|   Microchip Technology Inc.
|   PolarFire IBIS Model
[IBIS ver]   5.0
[File name]   polarfire_gpio_se.ibs
[File Rev]   2.3
[Date]   Wed Nov 22 2023
[Source] Simulated Models ONLY.
   All data is based on Spice simulation. All performed at Microchip Technology Inc.
[Notes]   This IBIS file is for GPIO single ended standards.
   Please refer to polarfire_gpio_diff.ibs for GPIO differential Standards Configurations,
   and refer to polarfire_hsio_se.ibs and polarfire_hsio_diff.ibs for HSIO Configurations.
   The package parasitics of various package types are given.
   Uncomment the appropriate package before simulations
   Revision History
   Rev 2.3: 22-Nov-2023
   - Added mixed mode receiver support:
   - Input buffers: LVCMOS12_15_CL_ODT-120,LVCMOS12_18_CL_ODT-120,LVCMOS12_25_CL_ODT-120,
   LVCMOS12_15_CL_ODT-240,LVCMOS12_18_CL_ODT-240,LVCMOS12_25_CL_ODT-240,
   LVCMOS18_15_ODT-120,LVCMOS18_25_ODT-120,LVCMOS18_15_ODT-240,LVCMOS18_25_ODT-240,
   HSUL18_33_ODT-OFF,HSUL18_25_ODT-OFF,HSUL18_15_ODT-OFF,HSUL18_12_ODT-OFF,
   HSUL18_ODT-OFF,HSUL18_ODT-50
   Rev 2.2: 26-Jul-2022
   - Vmeas_rising and Vmeas_falling of pci driver updated for more accuracy
   Rev 2.1: 4-May-2022
   - Vref_falling max voltage updated for pci driver
   - Added MPF050 device with RLC package data in [Package] section
   - Added RLC package type of FCG784N for MPF300T/TS device
   - Update RLC values of 200T-FCVG484 device package data
[Disclaimer] This information is for board design considerations.
   Simulation based V/I curves contained in this model file are
   considered preliminary until verified against bench
   measurements. Maximum currents may vary from part to part but
   should not exceed maximum I/V curves provided in this model file.
[Copyright]  (c) 2023, Microchip Technology Inc., All Rights Reserved.
| ADDITIONAL NOTES
|For Low Power Mobile Industry Processor Interface (MIPI) configuration,please use LVCMOS12 receiver IBIS models.
|Warnings for ISSO Pullup, Pulldown currents being non-zero maybe ignored.
|The naming conventions used in the signal_name/model_name are as follows:
| SLEW-#  - Slew setting,OFF or ON represented by #
| HYST-#  - Hysteresis setting,OFF or ON represented by #
| #mA   - Driver current strength, value represented by #
| #ohm   - Driver impedance mode, value represented by #
| ODT-#   - Series on-die termination, impedance value represented by #
| CL   - Receiver standards with clamp ON
| C1   - Refers to Class-I driver models
| C2   - Refers to Class-II driver models
| #_I   - Refers to input models ,  model name represented by #
| #_O   - Refers to output models , model name represented by #
| IBIS MODEL CHECKLIST
| Microchip Technology Inc. is dedicated to releasing quality IBIS models to customers.
| The following items have been
| verified for this IBIS model before release:
| 1)  Checked IBIS model by the golden parser ibischk5 [Complete]
| 2)  Ensured no errors reported by golden parser
|   for the IBIS model [Complete]
| 3)  Defined Vinl and Vinh for receivers [Complete]
| 4)  Defined Standard Load and Vmeas values for drivers [Complete]
| 5)  Defined overshoots for drivers and receivers [NA]
| 6)  Validated Ramp Values[]
| 7)  Defined V-T Tables for all output drivers [Complete]
| 8)  Validated [Diff Pins] [NA]
| 9)  Verified Package Parasitics [Complete]
| 10) Defined Standard Load Parameters and Specifications
|   for waveforms [Complete]
| 11) Defined and Validate Pin mappings [Complete]
| 12) Verified C_comp_pullup and C_comp_pulldown Values []
| 13) Visually Inspected I-V Curves and V-T Tables  [Complete]
| 14) Presented Typ/Min/Max Values in the correct order for
|   all tables and parameters [Complete]
| 15) Simulated all output models with standard load and
|   switching through Vmeas [Complete]
| 16) Simulated all receiver models  [Complete]
| 17) Validated Models selectors. [NA]
| 18) Visually inspected Spice and IBIS correlation for
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[Component]   PolarFire
[Manufacturer]   Microchip Technology Inc.
[Package]
|   typ   min   max
|MPF050T/TL/TLS/TS
|R_pkg   0.342   NA   NA   | MPF050T/TL/TLS/TS-FCSG325
|L_pkg   2.917nH   NA   NA   | MPF050T/TL/TLS/TS-FCSG325
|C_pkg   1.401pF   NA   NA   | MPF050T/TL/TLS/TS-FCSG325
|R_pkg   0.668   NA   NA   | MPF050T/TL/TLS/TS-FCVG484
|L_pkg   4.858nH   NA   NA   | MPF050T/TL/TLS/TS-FCVG484
|C_pkg   1.717pF   NA   NA   | MPF050T/TL/TLS/TS-FCVG484
|MPF100T/TL/TLS/TS
|R_pkg   0.277   NA   NA   | MPF100T/TL/TLS/TS-FCSG325
|L_pkg   2.866nH   NA   NA   | MPF100T/TL/TLS/TS-FCSG325
|C_pkg   0.601pF   NA   NA   | MPF100T/TL/TLS/TS-FCSG325
|R_pkg   0.960   NA   NA   | MPF100T/TL/TLS/TS-FCG484
|L_pkg   6.090nH   NA   NA   | MPF100T/TL/TLS/TS-FCG484
|C_pkg   2.182pF   NA   NA   | MPF100T/TL/TLS/TS-FCG484
|R_pkg   0.639   NA   NA   | MPF100T/TL/TLS/TS-FCVG484
|L_pkg   4.241nH   NA   NA   | MPF100T/TL/TLS/TS-FCVG484
|C_pkg   1.595pF   NA   NA   | MPF100T/TL/TLS/TS-FCVG484
|MPF200T/TL/TLS/TS
|R_pkg   0.392   NA   NA   | MPF200T/TL/TLS/TS-FCSG325
|L_pkg   3.035nH   NA   NA   | MPF200T/TL/TLS/TS-FCSG325
|C_pkg   0.970pF   NA   NA   | MPF200T/TL/TLS/TS-FCSG325
|R_pkg   0.885   NA   NA   | MPF200T/TL/TLS/TS-FCG484
|L_pkg   5.836nH   NA   NA   | MPF200T/TL/TLS/TS-FCG484
|C_pkg   2.013pF   NA   NA   | MPF200T/TL/TLS/TS-FCG484
|R_pkg   0.634   NA   NA   | MPF200T/TL/TLS/TS-FCVG484
|L_pkg   4.221nH   NA   NA   | MPF200T/TL/TLS/TS-FCVG484
|C_pkg   1.605pF   NA   NA   | MPF200T/TL/TLS/TS-FCVG484
|R_pkg   0.483   NA   NA   | MPF200T/TL/TLS/TS-FCSG536
|L_pkg   4.073nH   NA   NA   | MPF200T/TL/TLS/TS-FCSG536
|C_pkg   1.335pF   NA   NA   | MPF200T/TL/TLS/TS-FCSG536
|R_pkg   1.512   NA   NA   | MPF200T/TL/TLS/TS-FCG784
|L_pkg   9.182nH   NA   NA   | MPF200T/TL/TLS/TS-FCG784
|C_pkg   3.029pF   NA   NA   | MPF200T/TL/TLS/TS-FCG784
|MPF300T/TL/TLS/TS
|R_pkg   0.678   NA   NA   | MPF300T/TL/TLS/TS-FCG484
|L_pkg   5.038nH   NA   NA   | MPF300T/TL/TLS/TS-FCG484
|C_pkg   1.584pF   NA   NA   | MPF300T/TL/TLS/TS-FCG484
|R_pkg   0.702   NA   NA   | MPF300T/TL/TLS/TS-FCVG484
|L_pkg   4.503nH   NA   NA   | MPF300T/TL/TLS/TS-FCVG484
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R_pkg   1.478   NA   NA   | MPF300T/TL/TLS/TS-FCG1152
L_pkg   8.879nH   NA   NA   | MPF300T/TL/TLS/TS-FCG1152
C_pkg   2.839pF   NA   NA   | MPF300T/TL/TLS/TS-FCG1152
|MPF500T/TL/TLS/TS
|R_pkg   1.081   NA   NA   | MPF500T/TL/TLS/TS-FCG784
|L_pkg   6.727nH   NA   NA   | MPF500T/TL/TLS/TS-FCG784
|C_pkg   2.413pF   NA   NA   | MPF500T/TL/TLS/TS-FCG784
|R_pkg   1.419   NA   NA   | MPF500T/TL/TLS/TS-FCG1152
|L_pkg   8.917nH   NA   NA   | MPF500T/TL/TLS/TS-FCG1152
|C_pkg   2.924pF   NA   NA   | MPF500T/TL/TLS/TS-FCG1152
| End Header
| The PIN numbers given below are examples. They do not correspond to
| device pin numbers.
[Pin]   signal_name   model_name   R_pin   L_pin   C_pin
1   PCI_20mA_SLEW-ON_O   PCI_20mA_SLEW-ON_GPIO_O
2   PCI_20mA_SLEW-OFF_O   PCI_20mA_SLEW-OFF_GPIO_O
3   LVTTL_8mA_SLEW-ON_O   LVTTL_8mA_SLEW-ON_GPIO_O
4   LVTTL_8mA_SLEW-OFF_O   LVTTL_8mA_SLEW-OFF_GPIO_O
5   LVTTL_2mA_SLEW-ON_O   LVTTL_2mA_SLEW-ON_GPIO_O
6   LVTTL_2mA_SLEW-OFF_O   LVTTL_2mA_SLEW-OFF_GPIO_O
7   LVTTL_4mA_SLEW-ON_O   LVTTL_4mA_SLEW-ON_GPIO_O
8   LVTTL_4mA_SLEW-OFF_O   LVTTL_4mA_SLEW-OFF_GPIO_O
9   LVTTL_12mA_SLEW-ON_O   LVTTL_12mA_SLEW-ON_GPIO_O
10   LVTTL_12mA_SLEW-OFF_O   LVTTL_12mA_SLEW-OFF_GPIO_O
11   LVTTL_16mA_SLEW-ON_O   LVTTL_16mA_SLEW-ON_GPIO_O
12   LVTTL_16mA_SLEW-OFF_O   LVTTL_16mA_SLEW-OFF_GPIO_O
13   LVTTL_20mA_SLEW-ON_O   LVTTL_20mA_SLEW-ON_GPIO_O
14   LVTTL_20mA_SLEW-OFF_O   LVTTL_20mA_SLEW-OFF_GPIO_O
15   LVCMOS33_8mA_SLEW-ON_O   LVCMOS33_8mA_SLEW-ON_GPIO_O
16   LVCMOS33_8mA_SLEW-OFF_O   LVCMOS33_8mA_SLEW-OFF_GPIO_O
17   LVCMOS33_2mA_SLEW-ON_O   LVCMOS33_2mA_SLEW-ON_GPIO_O
18   LVCMOS33_2mA_SLEW-OFF_O   LVCMOS33_2mA_SLEW-OFF_GPIO_O
19   LVCMOS33_4mA_SLEW-ON_O   LVCMOS33_4mA_SLEW-ON_GPIO_O
20   LVCMOS33_4mA_SLEW-OFF_O   LVCMOS33_4mA_SLEW-OFF_GPIO_O
21   LVCMOS33_12mA_SLEW-ON_O   LVCMOS33_12mA_SLEW-ON_GPIO_O
22   LVCMOS33_12mA_SLEW-OFF_O   LVCMOS33_12mA_SLEW-OFF_GPIO_O
23   LVCMOS33_16mA_SLEW-ON_O   LVCMOS33_16mA_SLEW-ON_GPIO_O
24   LVCMOS33_16mA_SLEW-OFF_O   LVCMOS33_16mA_SLEW-OFF_GPIO_O
25   LVCMOS33_20mA_SLEW-ON_O   LVCMOS33_20mA_SLEW-ON_GPIO_O
26   LVCMOS33_20mA_SLEW-OFF_O   LVCMOS33_20mA_SLEW-OFF_GPIO_O
27   LVCMOS25_8mA_SLEW-ON_O   LVCMOS25_8mA_SLEW-ON_GPIO_O
28   LVCMOS25_8mA_SLEW-OFF_O   LVCMOS25_8mA_SLEW-OFF_GPIO_O
29   LVCMOS25_2mA_SLEW-ON_O   LVCMOS25_2mA_SLEW-ON_GPIO_O
30   LVCMOS25_2mA_SLEW-OFF_O   LVCMOS25_2mA_SLEW-OFF_GPIO_O
31   LVCMOS25_4mA_SLEW-ON_O   LVCMOS25_4mA_SLEW-ON_GPIO_O
32   LVCMOS25_4mA_SLEW-OFF_O   LVCMOS25_4mA_SLEW-OFF_GPIO_O
33   LVCMOS25_6mA_SLEW-ON_O   LVCMOS25_6mA_SLEW-ON_GPIO_O
34   LVCMOS25_6mA_SLEW-OFF_O   LVCMOS25_6mA_SLEW-OFF_GPIO_O
35   LVCMOS25_12mA_SLEW-ON_O   LVCMOS25_12mA_SLEW-ON_GPIO_O
36   LVCMOS25_12mA_SLEW-OFF_O   LVCMOS25_12mA_SLEW-OFF_GPIO_O
37   LVCMOS25_16mA_SLEW-ON_O   LVCMOS25_16mA_SLEW-ON_GPIO_O
38   LVCMOS25_16mA_SLEW-OFF_O   LVCMOS25_16mA_SLEW-OFF_GPIO_O
39   LVCMOS18_8mA_SLEW-OFF_O   LVCMOS18_8mA_SLEW-OFF_GPIO_O
40   LVCMOS18_2mA_SLEW-OFF_O   LVCMOS18_2mA_SLEW-OFF_GPIO_O
41   LVCMOS18_4mA_SLEW-OFF_O   LVCMOS18_4mA_SLEW-OFF_GPIO_O
42   LVCMOS18_6mA_SLEW-OFF_O   LVCMOS18_6mA_SLEW-OFF_GPIO_O
43   LVCMOS18_10mA_SLEW-OFF_O   LVCMOS18_10mA_SLEW-OFF_GPIO_O
44   LVCMOS18_12mA_SLEW-OFF_O   LVCMOS18_12mA_SLEW-OFF_GPIO_O
45   LVCMOS15_8mA_SLEW-OFF_O   LVCMOS15_8mA_SLEW-OFF_GPIO_O
46   LVCMOS15_2mA_SLEW-OFF_O   LVCMOS15_2mA_SLEW-OFF_GPIO_O
47   LVCMOS15_4mA_SLEW-OFF_O   LVCMOS15_4mA_SLEW-OFF_GPIO_O
48   LVCMOS15_6mA_SLEW-OFF_O   LVCMOS15_6mA_SLEW-OFF_GPIO_O
49   LVCMOS15_10mA_SLEW-OFF_O   LVCMOS15_10mA_SLEW-OFF_GPIO_O
50   LVCMOS12_8mA_SLEW-OFF_O   LVCMOS12_8mA_SLEW-OFF_GPIO_O
51   LVCMOS12_2mA_SLEW-OFF_O   LVCMOS12_2mA_SLEW-OFF_GPIO_O
52   LVCMOS12_4mA_SLEW-OFF_O   LVCMOS12_4mA_SLEW-OFF_GPIO_O
53   LVCMOS12_6mA_SLEW-OFF_O   LVCMOS12_6mA_SLEW-OFF_GPIO_O
54   SSTL25_C1_80ohm_SLEW-OFF_O   SSTL25_C1_80ohm_SLEW-OFF_GPIO_O
55   SSTL25_C1_120ohm_SLEW-OFF_O   SSTL25_C1_120ohm_SLEW-OFF_GPIO_O
56   SSTL25_C1_60ohm_SLEW-OFF_O   SSTL25_C1_60ohm_SLEW-OFF_GPIO_O
57   SSTL25_C1_48ohm_SLEW-OFF_O   SSTL25_C1_48ohm_SLEW-OFF_GPIO_O
58   SSTL25_C2_48ohm_SLEW-OFF_O   SSTL25_C2_48ohm_SLEW-OFF_GPIO_O
59   SSTL25_C2_60ohm_SLEW-OFF_O   SSTL25_C2_60ohm_SLEW-OFF_GPIO_O
60   SSTL25_C2_40ohm_SLEW-OFF_O   SSTL25_C2_40ohm_SLEW-OFF_GPIO_O
61   SSTL25_C2_34ohm_SLEW-OFF_O   SSTL25_C2_34ohm_SLEW-OFF_GPIO_O
62   SSTL18_C1_60ohm_SLEW-OFF_O   SSTL18_C1_60ohm_SLEW-OFF_GPIO_O
63   SSTL18_C1_80ohm_SLEW-OFF_O   SSTL18_C1_80ohm_SLEW-OFF_GPIO_O
64   SSTL18_C1_48ohm_SLEW-OFF_O   SSTL18_C1_48ohm_SLEW-OFF_GPIO_O
65   SSTL18_C1_40ohm_SLEW-OFF_O   SSTL18_C1_40ohm_SLEW-OFF_GPIO_O
66   SSTL18_C2_40ohm_SLEW-OFF_O   SSTL18_C2_40ohm_SLEW-OFF_GPIO_O
67   SSTL18_C2_48ohm_SLEW-OFF_O   SSTL18_C2_48ohm_SLEW-OFF_GPIO_O
68   SSTL18_C2_34ohm_SLEW-OFF_O   SSTL18_C2_34ohm_SLEW-OFF_GPIO_O
69   SSTL18_C2_30ohm_SLEW-OFF_O   SSTL18_C2_30ohm_SLEW-OFF_GPIO_O
70   SSTL15_C1_40ohm_SLEW-OFF_O   SSTL15_C1_40ohm_SLEW-OFF_GPIO_O
71   SSTL15_C1_48ohm_SLEW-OFF_O   SSTL15_C1_48ohm_SLEW-OFF_GPIO_O
72   SSTL15_C2_34ohm_SLEW-OFF_O   SSTL15_C2_34ohm_SLEW-OFF_GPIO_O
73   SSTL15_C2_30ohm_SLEW-OFF_O   SSTL15_C2_30ohm_SLEW-OFF_GPIO_O
74   SSTL15_C2_27ohm_SLEW-OFF_O   SSTL15_C2_27ohm_SLEW-OFF_GPIO_O
75   HSUL18_C1_55ohm_SLEW-OFF_O   HSUL18_C1_55ohm_SLEW-OFF_GPIO_O
76   HSUL18_C1_60ohm_SLEW-OFF_O   HSUL18_C1_60ohm_SLEW-OFF_GPIO_O
77   HSUL18_C1_40ohm_SLEW-OFF_O   HSUL18_C1_40ohm_SLEW-OFF_GPIO_O
78   HSUL18_C1_34ohm_SLEW-OFF_O   HSUL18_C1_34ohm_SLEW-OFF_GPIO_O
79   HSUL18_C2_25ohm_SLEW-OFF_O   HSUL18_C2_25ohm_SLEW-OFF_GPIO_O
80   HSUL18_C2_30ohm_SLEW-OFF_O   HSUL18_C2_30ohm_SLEW-OFF_GPIO_O
81   HSUL18_C2_27ohm_SLEW-OFF_O   HSUL18_C2_27ohm_SLEW-OFF_GPIO_O
82   HSUL18_C2_22ohm_SLEW-OFF_O   HSUL18_C2_22ohm_SLEW-OFF_GPIO_O
83   HSTL15_C1_50ohm_SLEW-OFF_O   HSTL15_C1_50ohm_SLEW-OFF_GPIO_O
84   HSTL15_C1_60ohm_SLEW-OFF_O   HSTL15_C1_60ohm_SLEW-OFF_GPIO_O
85   HSTL15_C1_40ohm_SLEW-OFF_O   HSTL15_C1_40ohm_SLEW-OFF_GPIO_O
86   HSTL15_C1_34ohm_SLEW-OFF_O   HSTL15_C1_34ohm_SLEW-OFF_GPIO_O
87   HSTL15_C2_25ohm_SLEW-OFF_O   HSTL15_C2_25ohm_SLEW-OFF_GPIO_O
88   HSTL15_C2_30ohm_SLEW-OFF_O   HSTL15_C2_30ohm_SLEW-OFF_GPIO_O
89   HSTL15_C2_27ohm_SLEW-OFF_O   HSTL15_C2_27ohm_SLEW-OFF_GPIO_O
90   HSTL15_C2_22ohm_SLEW-OFF_O   HSTL15_C2_22ohm_SLEW-OFF_GPIO_O
91   PCI_CL_ODT-OFF_HYST-ON_I   PCI_CL_ODT-OFF_HYST-ON_GPIO_I
92   PCI_CL_ODT-OFF_HYST-OFF_I   PCI_CL_ODT-OFF_HYST-OFF_GPIO_I
93   LVTTL_25_ODT-OFF_HYST-ON_I   LVTTL_25_ODT-OFF_HYST-ON_GPIO_I
94   LVTTL_18_ODT-OFF_HYST-ON_I   LVTTL_18_ODT-OFF_HYST-ON_GPIO_I
95   LVTTL_15_ODT-OFF_HYST-ON_I   LVTTL_15_ODT-OFF_HYST-ON_GPIO_I
96   LVTTL_12_ODT-OFF_HYST-ON_I   LVTTL_12_ODT-OFF_HYST-ON_GPIO_I
97   LVTTL_25_ODT-OFF_HYST-OFF_I   LVTTL_25_ODT-OFF_HYST-OFF_GPIO_I
98   LVTTL_18_ODT-OFF_HYST-OFF_I   LVTTL_18_ODT-OFF_HYST-OFF_GPIO_I
99   LVTTL_15_ODT-OFF_HYST-OFF_I   LVTTL_15_ODT-OFF_HYST-OFF_GPIO_I
100   LVTTL_12_ODT-OFF_HYST-OFF_I   LVTTL_12_ODT-OFF_HYST-OFF_GPIO_I
101   LVTTL_ODT-OFF_HYST-ON_I   LVTTL_ODT-OFF_HYST-ON_GPIO_I
102   LVTTL_ODT-OFF_HYST-OFF_I   LVTTL_ODT-OFF_HYST-OFF_GPIO_I
103   LVTTL_CL_ODT-OFF_HYST-ON_I   LVTTL_CL_ODT-OFF_HYST-ON_GPIO_I
104   LVTTL_CL_ODT-OFF_HYST-OFF_I   LVTTL_CL_ODT-OFF_HYST-OFF_GPIO_I
105   LVCMOS33_25_ODT-OFF_HYST-ON_I   LVCMOS33_25_ODT-OFF_HYST-ON_GPIO_I
106   LVCMOS33_18_ODT-OFF_HYST-ON_I   LVCMOS33_18_ODT-OFF_HYST-ON_GPIO_I
107   LVCMOS33_15_ODT-OFF_HYST-ON_I   LVCMOS33_15_ODT-OFF_HYST-ON_GPIO_I
108   LVCMOS33_12_ODT-OFF_HYST-ON_I   LVCMOS33_12_ODT-OFF_HYST-ON_GPIO_I
109   LVCMOS33_25_ODT-OFF_HYST-OFF_I   LVCMOS33_25_ODT-OFF_HYST-OFF_GPIO_I
110   LVCMOS33_18_ODT-OFF_HYST-OFF_I   LVCMOS33_18_ODT-OFF_HYST-OFF_GPIO_I
111   LVCMOS33_15_ODT-OFF_HYST-OFF_I   LVCMOS33_15_ODT-OFF_HYST-OFF_GPIO_I
112   LVCMOS33_12_ODT-OFF_HYST-OFF_I   LVCMOS33_12_ODT-OFF_HYST-OFF_GPIO_I
113   LVCMOS33_ODT-OFF_HYST-ON_I   LVCMOS33_ODT-OFF_HYST-ON_GPIO_I
114   LVCMOS33_ODT-OFF_HYST-OFF_I   LVCMOS33_ODT-OFF_HYST-OFF_GPIO_I
115   LVCMOS33_CL_ODT-OFF_HYST-ON_I   LVCMOS33_CL_ODT-OFF_HYST-ON_GPIO_I
116   LVCMOS33_CL_ODT-OFF_HYST-OFF_I   LVCMOS33_CL_ODT-OFF_HYST-OFF_GPIO_I
117   LVCMOS25_33_CL_ODT-OFF_HYST-ON_I   LVCMOS25_33_CL_ODT-OFF_HYST-ON_GPIO_I
118   LVCMOS25_33_CL_ODT-OFF_HYST-OFF_I   LVCMOS25_33_CL_ODT-OFF_HYST-OFF_GPIO_I
119   LVCMOS25_CL_ODT-OFF_HYST-ON_I   LVCMOS25_CL_ODT-OFF_HYST-ON_GPIO_I
120   LVCMOS25_CL_ODT-OFF_HYST-OFF_I   LVCMOS25_CL_ODT-OFF_HYST-OFF_GPIO_I
121   LVCMOS25_CL_ODT-120_HYST-ON_I   LVCMOS25_CL_ODT-120_HYST-ON_GPIO_I
122   LVCMOS25_CL_ODT-120_HYST-OFF_I   LVCMOS25_CL_ODT-120_HYST-OFF_GPIO_I
123   LVCMOS25_33_ODT-OFF_HYST-ON_I   LVCMOS25_33_ODT-OFF_HYST-ON_GPIO_I
124   LVCMOS25_33_ODT-OFF_HYST-OFF_I   LVCMOS25_33_ODT-OFF_HYST-OFF_GPIO_I
125   LVCMOS25_18_ODT-OFF_HYST-ON_I   LVCMOS25_18_ODT-OFF_HYST-ON_GPIO_I
126   LVCMOS25_15_ODT-OFF_HYST-ON_I   LVCMOS25_15_ODT-OFF_HYST-ON_GPIO_I
127   LVCMOS25_12_ODT-OFF_HYST-ON_I   LVCMOS25_12_ODT-OFF_HYST-ON_GPIO_I
128   LVCMOS25_18_ODT-OFF_HYST-OFF_I   LVCMOS25_18_ODT-OFF_HYST-OFF_GPIO_I
129   LVCMOS25_15_ODT-OFF_HYST-OFF_I   LVCMOS25_15_ODT-OFF_HYST-OFF_GPIO_I
130   LVCMOS25_12_ODT-OFF_HYST-OFF_I   LVCMOS25_12_ODT-OFF_HYST-OFF_GPIO_I
131   LVCMOS25_18_ODT-120_HYST-ON_I   LVCMOS25_18_ODT-120_HYST-ON_GPIO_I
132   LVCMOS25_15_ODT-120_HYST-ON_I   LVCMOS25_15_ODT-120_HYST-ON_GPIO_I
133   LVCMOS25_12_ODT-120_HYST-ON_I   LVCMOS25_12_ODT-120_HYST-ON_GPIO_I
134   LVCMOS25_18_ODT-120_HYST-OFF_I   LVCMOS25_18_ODT-120_HYST-OFF_GPIO_I
135   LVCMOS25_15_ODT-120_HYST-OFF_I   LVCMOS25_15_ODT-120_HYST-OFF_GPIO_I
136   LVCMOS25_12_ODT-120_HYST-OFF_I   LVCMOS25_12_ODT-120_HYST-OFF_GPIO_I
137   LVCMOS25_ODT-OFF_HYST-ON_I   LVCMOS25_ODT-OFF_HYST-ON_GPIO_I
138   LVCMOS25_ODT-OFF_HYST-OFF_I   LVCMOS25_ODT-OFF_HYST-OFF_GPIO_I
139   LVCMOS25_ODT-120_HYST-ON_I   LVCMOS25_ODT-120_HYST-ON_GPIO_I
140   LVCMOS25_ODT-120_HYST-OFF_I   LVCMOS25_ODT-120_HYST-OFF_GPIO_I
141   LVCMOS18_33_CL_ODT-OFF_HYST-OFF_I   LVCMOS18_33_CL_ODT-OFF_HYST-OFF_GPIO_I
142   LVCMOS18_25_CL_ODT-OFF_HYST-OFF_I   LVCMOS18_25_CL_ODT-OFF_HYST-OFF_GPIO_I
143   LVCMOS18_25_CL_ODT-120_HYST-OFF_I   LVCMOS18_25_CL_ODT-120_HYST-OFF_GPIO_I
144   LVCMOS18_25_CL_ODT-240_HYST-OFF_I   LVCMOS18_25_CL_ODT-240_HYST-OFF_GPIO_I
145   LVCMOS18_CL_ODT-OFF_HYST-OFF_I   LVCMOS18_CL_ODT-OFF_HYST-OFF_GPIO_I
146   LVCMOS18_CL_ODT-120_HYST-OFF_I   LVCMOS18_CL_ODT-120_HYST-OFF_GPIO_I
147   LVCMOS18_CL_ODT-240_HYST-OFF_I   LVCMOS18_CL_ODT-240_HYST-OFF_GPIO_I
148   LVCMOS18_33_ODT-OFF_HYST-OFF_I   LVCMOS18_33_ODT-OFF_HYST-OFF_GPIO_I
149   LVCMOS18_25_ODT-OFF_HYST-OFF_I   LVCMOS18_25_ODT-OFF_HYST-OFF_GPIO_I
150   LVCMOS18_15_ODT-OFF_HYST-OFF_I   LVCMOS18_15_ODT-OFF_HYST-OFF_GPIO_I
151   LVCMOS18_ODT-OFF_HYST-OFF_I   LVCMOS18_ODT-OFF_HYST-OFF_GPIO_I
152   LVCMOS18_ODT-120_HYST-OFF_I   LVCMOS18_ODT-120_HYST-OFF_GPIO_I
153   LVCMOS18_ODT-240_HYST-OFF_I   LVCMOS18_ODT-240_HYST-OFF_GPIO_I
154   LVCMOS15_25_CL_ODT-OFF_HYST-OFF_I   LVCMOS15_25_CL_ODT-OFF_HYST-OFF_GPIO_I
155   LVCMOS15_18_CL_ODT-OFF_HYST-OFF_I   LVCMOS15_18_CL_ODT-OFF_HYST-OFF_GPIO_I
156   LVCMOS15_25_CL_ODT-120_HYST-OFF_I   LVCMOS15_25_CL_ODT-120_HYST-OFF_GPIO_I
157   LVCMOS15_18_CL_ODT-120_HYST-OFF_I   LVCMOS15_18_CL_ODT-120_HYST-OFF_GPIO_I
158   LVCMOS15_25_CL_ODT-240_HYST-OFF_I   LVCMOS15_25_CL_ODT-240_HYST-OFF_GPIO_I
159   LVCMOS15_18_CL_ODT-240_HYST-OFF_I   LVCMOS15_18_CL_ODT-240_HYST-OFF_GPIO_I
160   LVCMOS15_CL_ODT-OFF_HYST-OFF_I   LVCMOS15_CL_ODT-OFF_HYST-OFF_GPIO_I
161   LVCMOS15_CL_ODT-120_HYST-OFF_I   LVCMOS15_CL_ODT-120_HYST-OFF_GPIO_I
162   LVCMOS15_CL_ODT-240_HYST-OFF_I   LVCMOS15_CL_ODT-240_HYST-OFF_GPIO_I
163   LVCMOS15_25_ODT-OFF_HYST-OFF_I   LVCMOS15_25_ODT-OFF_HYST-OFF_GPIO_I
164   LVCMOS15_18_ODT-OFF_HYST-OFF_I   LVCMOS15_18_ODT-OFF_HYST-OFF_GPIO_I
165   LVCMOS15_12_ODT-OFF_HYST-OFF_I   LVCMOS15_12_ODT-OFF_HYST-OFF_GPIO_I
166   LVCMOS15_25_ODT-120_HYST-OFF_I   LVCMOS15_25_ODT-120_HYST-OFF_GPIO_I
167   LVCMOS15_18_ODT-120_HYST-OFF_I   LVCMOS15_18_ODT-120_HYST-OFF_GPIO_I
168   LVCMOS15_12_ODT-120_HYST-OFF_I   LVCMOS15_12_ODT-120_HYST-OFF_GPIO_I
169   LVCMOS15_25_ODT-240_HYST-OFF_I   LVCMOS15_25_ODT-240_HYST-OFF_GPIO_I
170   LVCMOS15_18_ODT-240_HYST-OFF_I   LVCMOS15_18_ODT-240_HYST-OFF_GPIO_I
171   LVCMOS15_12_ODT-240_HYST-OFF_I   LVCMOS15_12_ODT-240_HYST-OFF_GPIO_I
172   LVCMOS15_ODT-OFF_HYST-OFF_I   LVCMOS15_ODT-OFF_HYST-OFF_GPIO_I
173   LVCMOS15_ODT-120_HYST-OFF_I   LVCMOS15_ODT-120_HYST-OFF_GPIO_I
174   LVCMOS15_ODT-240_HYST-OFF_I   LVCMOS15_ODT-240_HYST-OFF_GPIO_I
175   LVCMOS12_33_CL_ODT-OFF_HYST-OFF_I   LVCMOS12_33_CL_ODT-OFF_HYST-OFF_GPIO_I
176   LVCMOS12_25_CL_ODT-OFF_HYST-OFF_I   LVCMOS12_25_CL_ODT-OFF_HYST-OFF_GPIO_I
177   LVCMOS12_18_CL_ODT-OFF_HYST-OFF_I   LVCMOS12_18_CL_ODT-OFF_HYST-OFF_GPIO_I
178   LVCMOS12_15_CL_ODT-OFF_HYST-OFF_I   LVCMOS12_15_CL_ODT-OFF_HYST-OFF_GPIO_I
179   LVCMOS12_CL_ODT-OFF_HYST-OFF_I   LVCMOS12_CL_ODT-OFF_HYST-OFF_GPIO_I
180   LVCMOS12_CL_ODT-120_HYST-OFF_I   LVCMOS12_CL_ODT-120_HYST-OFF_GPIO_I
181   LVCMOS12_CL_ODT-240_HYST-OFF_I   LVCMOS12_CL_ODT-240_HYST-OFF_GPIO_I
182   LVCMOS12_33_ODT-OFF_HYST-OFF_I   LVCMOS12_33_ODT-OFF_HYST-OFF_GPIO_I
183   LVCMOS12_25_ODT-OFF_HYST-OFF_I   LVCMOS12_25_ODT-OFF_HYST-OFF_GPIO_I
184   LVCMOS12_18_ODT-OFF_HYST-OFF_I   LVCMOS12_18_ODT-OFF_HYST-OFF_GPIO_I
185   LVCMOS12_15_ODT-OFF_HYST-OFF_I   LVCMOS12_15_ODT-OFF_HYST-OFF_GPIO_I
186   LVCMOS12_25_ODT-120_HYST-OFF_I   LVCMOS12_25_ODT-120_HYST-OFF_GPIO_I
187   LVCMOS12_18_ODT-120_HYST-OFF_I   LVCMOS12_18_ODT-120_HYST-OFF_GPIO_I
188   LVCMOS12_15_ODT-120_HYST-OFF_I   LVCMOS12_15_ODT-120_HYST-OFF_GPIO_I
189   LVCMOS12_25_ODT-240_HYST-OFF_I   LVCMOS12_25_ODT-240_HYST-OFF_GPIO_I
190   LVCMOS12_18_ODT-240_HYST-OFF_I   LVCMOS12_18_ODT-240_HYST-OFF_GPIO_I
191   LVCMOS12_15_ODT-240_HYST-OFF_I   LVCMOS12_15_ODT-240_HYST-OFF_GPIO_I
192   LVCMOS12_ODT-OFF_HYST-OFF_I   LVCMOS12_ODT-OFF_HYST-OFF_GPIO_I
193   LVCMOS12_ODT-120_HYST-OFF_I   LVCMOS12_ODT-120_HYST-OFF_GPIO_I
194   LVCMOS12_ODT-240_HYST-OFF_I   LVCMOS12_ODT-240_HYST-OFF_GPIO_I
195   SSTL25_33_CL_ODT-OFF_HYST-OFF_I   SSTL25_33_CL_ODT-OFF_HYST-OFF_GPIO_I
196   SSTL25_CL_ODT-OFF_HYST-OFF_I   SSTL25_CL_ODT-OFF_HYST-OFF_GPIO_I
197   SSTL25_33_ODT-OFF_HYST-OFF_I   SSTL25_33_ODT-OFF_HYST-OFF_GPIO_I
198   SSTL25_ODT-OFF_HYST-OFF_I   SSTL25_ODT-OFF_HYST-OFF_GPIO_I
199   SSTL25_18_ODT-OFF_HYST-OFF_I   SSTL25_18_ODT-OFF_HYST-OFF_GPIO_I
200   SSTL25_15_ODT-OFF_HYST-OFF_I   SSTL25_15_ODT-OFF_HYST-OFF_GPIO_I
201   SSTL25_12_ODT-OFF_HYST-OFF_I   SSTL25_12_ODT-OFF_HYST-OFF_GPIO_I
202   SSTL18_33_CL_ODT-OFF_HYST-OFF_I   SSTL18_33_CL_ODT-OFF_HYST-OFF_GPIO_I
203   SSTL18_25_CL_ODT-OFF_HYST-OFF_I   SSTL18_25_CL_ODT-OFF_HYST-OFF_GPIO_I
204   SSTL18_CL_ODT-OFF_HYST-OFF_I   SSTL18_CL_ODT-OFF_HYST-OFF_GPIO_I
205   SSTL18_CL_ODT-50_HYST-OFF_I   SSTL18_CL_ODT-50_HYST-OFF_GPIO_I
206   SSTL18_CL_ODT-150_HYST-OFF_I   SSTL18_CL_ODT-150_HYST-OFF_GPIO_I
207   SSTL18_CL_ODT-75_HYST-OFF_I   SSTL18_CL_ODT-75_HYST-OFF_GPIO_I
208   SSTL18_33_ODT-OFF_HYST-OFF_I   SSTL18_33_ODT-OFF_HYST-OFF_GPIO_I
209   SSTL18_25_ODT-OFF_HYST-OFF_I   SSTL18_25_ODT-OFF_HYST-OFF_GPIO_I
210   SSTL18_15_ODT-OFF_HYST-OFF_I   SSTL18_15_ODT-OFF_HYST-OFF_GPIO_I
211   SSTL18_12_ODT-OFF_HYST-OFF_I   SSTL18_12_ODT-OFF_HYST-OFF_GPIO_I
212   SSTL18_ODT-OFF_HYST-OFF_I   SSTL18_ODT-OFF_HYST-OFF_GPIO_I
213   SSTL18_ODT-50_HYST-OFF_I   SSTL18_ODT-50_HYST-OFF_GPIO_I
214   SSTL18_ODT-150_HYST-OFF_I   SSTL18_ODT-150_HYST-OFF_GPIO_I
215   SSTL18_ODT-75_HYST-OFF_I   SSTL18_ODT-75_HYST-OFF_GPIO_I
216   SSTL15_33_CL_ODT-OFF_HYST-OFF_I   SSTL15_33_CL_ODT-OFF_HYST-OFF_GPIO_I
217   SSTL15_25_CL_ODT-OFF_HYST-OFF_I   SSTL15_25_CL_ODT-OFF_HYST-OFF_GPIO_I
218   SSTL15_18_CL_ODT-OFF_HYST-OFF_I   SSTL15_18_CL_ODT-OFF_HYST-OFF_GPIO_I
219   SSTL15_CL_ODT-OFF_HYST-OFF_I   SSTL15_CL_ODT-OFF_HYST-OFF_GPIO_I
220   SSTL15_CL_ODT-60_HYST-OFF_I   SSTL15_CL_ODT-60_HYST-OFF_GPIO_I
221   SSTL15_CL_ODT-120_HYST-OFF_I   SSTL15_CL_ODT-120_HYST-OFF_GPIO_I
222   SSTL15_CL_ODT-40_HYST-OFF_I   SSTL15_CL_ODT-40_HYST-OFF_GPIO_I
223   SSTL15_CL_ODT-30_HYST-OFF_I   SSTL15_CL_ODT-30_HYST-OFF_GPIO_I
224   SSTL15_CL_ODT-20_HYST-OFF_I   SSTL15_CL_ODT-20_HYST-OFF_GPIO_I
225   SSTL15_33_ODT-OFF_HYST-OFF_I   SSTL15_33_ODT-OFF_HYST-OFF_GPIO_I
226   SSTL15_25_ODT-OFF_HYST-OFF_I   SSTL15_25_ODT-OFF_HYST-OFF_GPIO_I
227   SSTL15_18_ODT-OFF_HYST-OFF_I   SSTL15_18_ODT-OFF_HYST-OFF_GPIO_I
228   SSTL15_12_ODT-OFF_HYST-OFF_I   SSTL15_12_ODT-OFF_HYST-OFF_GPIO_I
229   SSTL15_ODT-OFF_HYST-OFF_I   SSTL15_ODT-OFF_HYST-OFF_GPIO_I
230   SSTL15_ODT-60_HYST-OFF_I   SSTL15_ODT-60_HYST-OFF_GPIO_I
231   SSTL15_ODT-120_HYST-OFF_I   SSTL15_ODT-120_HYST-OFF_GPIO_I
232   SSTL15_ODT-40_HYST-OFF_I   SSTL15_ODT-40_HYST-OFF_GPIO_I
233   SSTL15_ODT-30_HYST-OFF_I   SSTL15_ODT-30_HYST-OFF_GPIO_I
234   SSTL15_ODT-20_HYST-OFF_I   SSTL15_ODT-20_HYST-OFF_GPIO_I
235   HSUL18_33_CL_ODT-OFF_HYST-OFF_I   HSUL18_33_CL_ODT-OFF_HYST-OFF_GPIO_I
236   HSUL18_25_CL_ODT-OFF_HYST-OFF_I   HSUL18_25_CL_ODT-OFF_HYST-OFF_GPIO_I
237   HSUL18_CL_ODT-OFF_HYST-OFF_I   HSUL18_CL_ODT-OFF_HYST-OFF_GPIO_I
238   HSUL18_CL_ODT-50_HYST-OFF_I   HSUL18_CL_ODT-50_HYST-OFF_GPIO_I
239   HSTL15_33_CL_ODT-OFF_HYST-OFF_I   HSTL15_33_CL_ODT-OFF_HYST-OFF_GPIO_I
240   HSTL15_25_CL_ODT-OFF_HYST-OFF_I   HSTL15_25_CL_ODT-OFF_HYST-OFF_GPIO_I
241   HSTL15_18_CL_ODT-OFF_HYST-OFF_I   HSTL15_18_CL_ODT-OFF_HYST-OFF_GPIO_I
242   HSTL15_CL_ODT-OFF_HYST-OFF_I   HSTL15_CL_ODT-OFF_HYST-OFF_GPIO_I
243   HSTL15_CL_ODT-50_HYST-OFF_I   HSTL15_CL_ODT-50_HYST-OFF_GPIO_I
244   HSTL15_33_ODT-OFF_HYST-OFF_I   HSTL15_33_ODT-OFF_HYST-OFF_GPIO_I
245   HSTL15_25_ODT-OFF_HYST-OFF_I   HSTL15_25_ODT-OFF_HYST-OFF_GPIO_I
246   HSTL15_18_ODT-OFF_HYST-OFF_I   HSTL15_18_ODT-OFF_HYST-OFF_GPIO_I
247   HSTL15_12_ODT-OFF_HYST-OFF_I   HSTL15_12_ODT-OFF_HYST-OFF_GPIO_I
248   HSTL15_ODT-OFF_HYST-OFF_I   HSTL15_ODT-OFF_HYST-OFF_GPIO_I
249   HSTL15_ODT-50_HYST-OFF_I   HSTL15_ODT-50_HYST-OFF_GPIO_I
250   LVCMOS12_25_CL_ODT-120_HYST-OFF_I   LVCMOS12_25_CL_ODT-120_HYST-OFF_GPIO_I
251   LVCMOS12_18_CL_ODT-120_HYST-OFF_I   LVCMOS12_18_CL_ODT-120_HYST-OFF_GPIO_I
252   LVCMOS12_15_CL_ODT-120_HYST-OFF_I   LVCMOS12_15_CL_ODT-120_HYST-OFF_GPIO_I
253   LVCMOS12_25_CL_ODT-240_HYST-OFF_I   LVCMOS12_25_CL_ODT-240_HYST-OFF_GPIO_I
254   LVCMOS12_18_CL_ODT-240_HYST-OFF_I   LVCMOS12_18_CL_ODT-240_HYST-OFF_GPIO_I
255   LVCMOS12_15_CL_ODT-240_HYST-OFF_I   LVCMOS12_15_CL_ODT-240_HYST-OFF_GPIO_I
256   LVCMOS18_15_ODT-120_HYST-OFF_I   LVCMOS18_15_ODT-120_HYST-OFF_GPIO_I
257   LVCMOS18_15_ODT-240_HYST-OFF_I   LVCMOS18_15_ODT-240_HYST-OFF_GPIO_I
258   LVCMOS18_25_ODT-120_HYST-OFF_I   LVCMOS18_25_ODT-120_HYST-OFF_GPIO_I
259   LVCMOS18_25_ODT-240_HYST-OFF_I   LVCMOS18_25_ODT-240_HYST-OFF_GPIO_I
260   HSUL18_33_ODT-OFF_HYST-OFF_I   HSUL18_33_ODT-OFF_HYST-OFF_GPIO_I
261   HSUL18_25_ODT-OFF_HYST-OFF_I   HSUL18_25_ODT-OFF_HYST-OFF_GPIO_I
262   HSUL18_15_ODT-OFF_HYST-OFF_I   HSUL18_15_ODT-OFF_HYST-OFF_GPIO_I
263   HSUL18_12_ODT-OFF_HYST-OFF_I   HSUL18_12_ODT-OFF_HYST-OFF_GPIO_I
264   HSUL18_ODT-OFF_HYST-OFF_I   HSUL18_ODT-OFF_HYST-OFF_GPIO_I
265   HSUL18_ODT-50_HYST-OFF_I   HSUL18_ODT-50_HYST-OFF_GPIO_I
266   VDDI   POWER
267   VSS   GND
[Pin Mapping]   pulldown_ref   pullup_ref   gnd_clamp_ref   power_clamp_ref   ext_ref
1   VSS   VDDI   VSS   VDDI
2   VSS   VDDI   VSS   VDDI
3   VSS   VDDI   VSS   VDDI
4   VSS   VDDI   VSS   VDDI
5   VSS   VDDI   VSS   VDDI
6   VSS   VDDI   VSS   VDDI
7   VSS   VDDI   VSS   VDDI
8   VSS   VDDI   VSS   VDDI
9   VSS   VDDI   VSS   VDDI
10   VSS   VDDI   VSS   VDDI
11   VSS   VDDI   VSS   VDDI
12   VSS   VDDI   VSS   VDDI
13   VSS   VDDI   VSS   VDDI
14   VSS   VDDI   VSS   VDDI
15   VSS   VDDI   VSS   VDDI
16   VSS   VDDI   VSS   VDDI
17   VSS   VDDI   VSS   VDDI
18   VSS   VDDI   VSS   VDDI
19   VSS   VDDI   VSS   VDDI
20   VSS   VDDI   VSS   VDDI
21   VSS   VDDI   VSS   VDDI
22   VSS   VDDI   VSS   VDDI
23   VSS   VDDI   VSS   VDDI
24   VSS   VDDI   VSS   VDDI
25   VSS   VDDI   VSS   VDDI
26   VSS   VDDI   VSS   VDDI
27   VSS   VDDI   VSS   VDDI
28   VSS   VDDI   VSS   VDDI
29   VSS   VDDI   VSS   VDDI
30   VSS   VDDI   VSS   VDDI
31   VSS   VDDI   VSS   VDDI
32   VSS   VDDI   VSS   VDDI
33   VSS   VDDI   VSS   VDDI
34   VSS   VDDI   VSS   VDDI
35   VSS   VDDI   VSS   VDDI
36   VSS   VDDI   VSS   VDDI
37   VSS   VDDI   VSS   VDDI
38   VSS   VDDI   VSS   VDDI
39   VSS   VDDI   VSS   VDDI
40   VSS   VDDI   VSS   VDDI
41   VSS   VDDI   VSS   VDDI
42   VSS   VDDI   VSS   VDDI
43   VSS   VDDI   VSS   VDDI
44   VSS   VDDI   VSS   VDDI
45   VSS   VDDI   VSS   VDDI
46   VSS   VDDI   VSS   VDDI
47   VSS   VDDI   VSS   VDDI
48   VSS   VDDI   VSS   VDDI
49   VSS   VDDI   VSS   VDDI
50   VSS   VDDI   VSS   VDDI
51   VSS   VDDI   VSS   VDDI
52   VSS   VDDI   VSS   VDDI
53   VSS   VDDI   VSS   VDDI
54   VSS   VDDI   VSS   VDDI
55   VSS   VDDI   VSS   VDDI
56   VSS   VDDI   VSS   VDDI
57   VSS   VDDI   VSS   VDDI
58   VSS   VDDI   VSS   VDDI
59   VSS   VDDI   VSS   VDDI
60   VSS   VDDI   VSS   VDDI
61   VSS   VDDI   VSS   VDDI
62   VSS   VDDI   VSS   VDDI
63   VSS   VDDI   VSS   VDDI
64   VSS   VDDI   VSS   VDDI
65   VSS   VDDI   VSS   VDDI
66   VSS   VDDI   VSS   VDDI
67   VSS   VDDI   VSS   VDDI
68   VSS   VDDI   VSS   VDDI
69   VSS   VDDI   VSS   VDDI
70   VSS   VDDI   VSS   VDDI
71   VSS   VDDI   VSS   VDDI
72   VSS   VDDI   VSS   VDDI
73   VSS   VDDI   VSS   VDDI
74   VSS   VDDI   VSS   VDDI
75   VSS   VDDI   VSS   VDDI
76   VSS   VDDI   VSS   VDDI
77   VSS   VDDI   VSS   VDDI
78   VSS   VDDI   VSS   VDDI
79   VSS   VDDI   VSS   VDDI
80   VSS   VDDI   VSS   VDDI
81   VSS   VDDI   VSS   VDDI
82   VSS   VDDI   VSS   VDDI
83   VSS   VDDI   VSS   VDDI
84   VSS   VDDI   VSS   VDDI
85   VSS   VDDI   VSS   VDDI
86   VSS   VDDI   VSS   VDDI
87   VSS   VDDI   VSS   VDDI
88   VSS   VDDI   VSS   VDDI
89   VSS   VDDI   VSS   VDDI
90   VSS   VDDI   VSS   VDDI
91   VSS   VDDI   VSS   VDDI
92   VSS   VDDI   VSS   VDDI
93   VSS   VDDI   VSS   VDDI
94   VSS   VDDI   VSS   VDDI
95   VSS   VDDI   VSS   VDDI
96   VSS   VDDI   VSS   VDDI
97   VSS   VDDI   VSS   VDDI
98   VSS   VDDI   VSS   VDDI
99   VSS   VDDI   VSS   VDDI
100   VSS   VDDI   VSS   VDDI
101   VSS   VDDI   VSS   VDDI
102   VSS   VDDI   VSS   VDDI
103   VSS   VDDI   VSS   VDDI
104   VSS   VDDI   VSS   VDDI
105   VSS   VDDI   VSS   VDDI
106   VSS   VDDI   VSS   VDDI
107   VSS   VDDI   VSS   VDDI
108   VSS   VDDI   VSS   VDDI
109   VSS   VDDI   VSS   VDDI
110   VSS   VDDI   VSS   VDDI
111   VSS   VDDI   VSS   VDDI
112   VSS   VDDI   VSS   VDDI
113   VSS   VDDI   VSS   VDDI
114   VSS   VDDI   VSS   VDDI
115   VSS   VDDI   VSS   VDDI
116   VSS   VDDI   VSS   VDDI
117   VSS   VDDI   VSS   VDDI
118   VSS   VDDI   VSS   VDDI
119   VSS   VDDI   VSS   VDDI
120   VSS   VDDI   VSS   VDDI
121   VSS   VDDI   VSS   VDDI
122   VSS   VDDI   VSS   VDDI
123   VSS   VDDI   VSS   VDDI
124   VSS   VDDI   VSS   VDDI
125   VSS   VDDI   VSS   VDDI
126   VSS   VDDI   VSS   VDDI
127   VSS   VDDI   VSS   VDDI
128   VSS   VDDI   VSS   VDDI
129   VSS   VDDI   VSS   VDDI
130   VSS   VDDI   VSS   VDDI
131   VSS   VDDI   VSS   VDDI
132   VSS   VDDI   VSS   VDDI
133   VSS   VDDI   VSS   VDDI
134   VSS   VDDI   VSS   VDDI
135   VSS   VDDI   VSS   VDDI
136   VSS   VDDI   VSS   VDDI
137   VSS   VDDI   VSS   VDDI
138   VSS   VDDI   VSS   VDDI
139   VSS   VDDI   VSS   VDDI
140   VSS   VDDI   VSS   VDDI
141   VSS   VDDI   VSS   VDDI
142   VSS   VDDI   VSS   VDDI
143   VSS   VDDI   VSS   VDDI
144   VSS   VDDI   VSS   VDDI
145   VSS   VDDI   VSS   VDDI
146   VSS   VDDI   VSS   VDDI
147   VSS   VDDI   VSS   VDDI
148   VSS   VDDI   VSS   VDDI
149   VSS   VDDI   VSS   VDDI
150   VSS   VDDI   VSS   VDDI
151   VSS   VDDI   VSS   VDDI
152   VSS   VDDI   VSS   VDDI
153   VSS   VDDI   VSS   VDDI
154   VSS   VDDI   VSS   VDDI
155   VSS   VDDI   VSS   VDDI
156   VSS   VDDI   VSS   VDDI
157   VSS   VDDI   VSS   VDDI
158   VSS   VDDI   VSS   VDDI
159   VSS   VDDI   VSS   VDDI
160   VSS   VDDI   VSS   VDDI
161   VSS   VDDI   VSS   VDDI
162   VSS   VDDI   VSS   VDDI
163   VSS   VDDI   VSS   VDDI
164   VSS   VDDI   VSS   VDDI
165   VSS   VDDI   VSS   VDDI
166   VSS   VDDI   VSS   VDDI
167   VSS   VDDI   VSS   VDDI
168   VSS   VDDI   VSS   VDDI
169   VSS   VDDI   VSS   VDDI
170   VSS   VDDI   VSS   VDDI
171   VSS   VDDI   VSS   VDDI
172   VSS   VDDI   VSS   VDDI
173   VSS   VDDI   VSS   VDDI
174   VSS   VDDI   VSS   VDDI
175   VSS   VDDI   VSS   VDDI
176   VSS   VDDI   VSS   VDDI
177   VSS   VDDI   VSS   VDDI
178   VSS   VDDI   VSS   VDDI
179   VSS   VDDI   VSS   VDDI
180   VSS   VDDI   VSS   VDDI
181   VSS   VDDI   VSS   VDDI
182   VSS   VDDI   VSS   VDDI
183   VSS   VDDI   VSS   VDDI
184   VSS   VDDI   VSS   VDDI
185   VSS   VDDI   VSS   VDDI
186   VSS   VDDI   VSS   VDDI
187   VSS   VDDI   VSS   VDDI
188   VSS   VDDI   VSS   VDDI
189   VSS   VDDI   VSS   VDDI
190   VSS   VDDI   VSS   VDDI
191   VSS   VDDI   VSS   VDDI
192   VSS   VDDI   VSS   VDDI
193   VSS   VDDI   VSS   VDDI
194   VSS   VDDI   VSS   VDDI
195   VSS   VDDI   VSS   VDDI
196   VSS   VDDI   VSS   VDDI
197   VSS   VDDI   VSS   VDDI
198   VSS   VDDI   VSS   VDDI
199   VSS   VDDI   VSS   VDDI
200   VSS   VDDI   VSS   VDDI
201   VSS   VDDI   VSS   VDDI
202   VSS   VDDI   VSS   VDDI
203   VSS   VDDI   VSS   VDDI
204   VSS   VDDI   VSS   VDDI
205   VSS   VDDI   VSS   VDDI
206   VSS   VDDI   VSS   VDDI
207   VSS   VDDI   VSS   VDDI
208   VSS   VDDI   VSS   VDDI
209   VSS   VDDI   VSS   VDDI
210   VSS   VDDI   VSS   VDDI
211   VSS   VDDI   VSS   VDDI
212   VSS   VDDI   VSS   VDDI
213   VSS   VDDI   VSS   VDDI
214   VSS   VDDI   VSS   VDDI
215   VSS   VDDI   VSS   VDDI
216   VSS   VDDI   VSS   VDDI
217   VSS   VDDI   VSS   VDDI
218   VSS   VDDI   VSS   VDDI
219   VSS   VDDI   VSS   VDDI
220   VSS   VDDI   VSS   VDDI
221   VSS   VDDI   VSS   VDDI
222   VSS   VDDI   VSS   VDDI
223   VSS   VDDI   VSS   VDDI
224   VSS   VDDI   VSS   VDDI
225   VSS   VDDI   VSS   VDDI
226   VSS   VDDI   VSS   VDDI
227   VSS   VDDI   VSS   VDDI
228   VSS   VDDI   VSS   VDDI
229   VSS   VDDI   VSS   VDDI
230   VSS   VDDI   VSS   VDDI
231   VSS   VDDI   VSS   VDDI
232   VSS   VDDI   VSS   VDDI
233   VSS   VDDI   VSS   VDDI
234   VSS   VDDI   VSS   VDDI
235   VSS   VDDI   VSS   VDDI
236   VSS   VDDI   VSS   VDDI
237   VSS   VDDI   VSS   VDDI
238   VSS   VDDI   VSS   VDDI
239   VSS   VDDI   VSS   VDDI
240   VSS   VDDI   VSS   VDDI
241   VSS   VDDI   VSS   VDDI
242   VSS   VDDI   VSS   VDDI
243   VSS   VDDI   VSS   VDDI
244   VSS   VDDI   VSS   VDDI
245   VSS   VDDI   VSS   VDDI
246   VSS   VDDI   VSS   VDDI
247   VSS   VDDI   VSS   VDDI
248   VSS   VDDI   VSS   VDDI
249   VSS   VDDI   VSS   VDDI
250   VSS   VDDI   VSS   VDDI
251   VSS   VDDI   VSS   VDDI
252   VSS   VDDI   VSS   VDDI
253   VSS   VDDI   VSS   VDDI
254   VSS   VDDI   VSS   VDDI
255   VSS   VDDI   VSS   VDDI
256   VSS   VDDI   VSS   VDDI
257   VSS   VDDI   VSS   VDDI
258   VSS   VDDI   VSS   VDDI
259   VSS   VDDI   VSS   VDDI
260   VSS   VDDI   VSS   VDDI
261   VSS   VDDI   VSS   VDDI
262   VSS   VDDI   VSS   VDDI
263   VSS   VDDI   VSS   VDDI
264   VSS   VDDI   VSS   VDDI
265   VSS   VDDI   VSS   VDDI
266   NC   VDDI
267   VSS   NC
| Models and submodels in the file (265): PCI_20mA_SLEW-ON_GPIO_O (Output), PCI_20mA_SLEW-OFF_GPIO_O (Output), LVTTL_8mA_SLEW-ON_GPIO_O (Output), LVTTL_8mA_SLEW-OFF_GPIO_O (Output), LVTTL_2mA_SLEW-ON_GPIO_O (Output), LVTTL_2mA_SLEW-OFF_GPIO_O (Output), LVTTL_4mA_SLEW-ON_GPIO_O (Output), LVTTL_4mA_SLEW-OFF_GPIO_O (Output), LVTTL_12mA_SLEW-ON_GPIO_O (Output), LVTTL_12mA_SLEW-OFF_GPIO_O (Output), LVTTL_16mA_SLEW-ON_GPIO_O (Output), LVTTL_16mA_SLEW-OFF_GPIO_O (Output), LVTTL_20mA_SLEW-ON_GPIO_O (Output), LVTTL_20mA_SLEW-OFF_GPIO_O (Output), LVCMOS33_8mA_SLEW-ON_GPIO_O (Output), LVCMOS33_8mA_SLEW-OFF_GPIO_O (Output), LVCMOS33_2mA_SLEW-ON_GPIO_O (Output), LVCMOS33_2mA_SLEW-OFF_GPIO_O (Output), LVCMOS33_4mA_SLEW-ON_GPIO_O (Output), LVCMOS33_4mA_SLEW-OFF_GPIO_O (Output), LVCMOS33_12mA_SLEW-ON_GPIO_O (Output), LVCMOS33_12mA_SLEW-OFF_GPIO_O (Output), LVCMOS33_16mA_SLEW-ON_GPIO_O (Output), LVCMOS33_16mA_SLEW-OFF_GPIO_O (Output), LVCMOS33_20mA_SLEW-ON_GPIO_O (Output), LVCMOS33_20mA_SLEW-OFF_GPIO_O (Output), LVCMOS25_8mA_SLEW-ON_GPIO_O (Output), LVCMOS25_8mA_SLEW-OFF_GPIO_O (Output), LVCMOS25_2mA_SLEW-ON_GPIO_O (Output), LVCMOS25_2mA_SLEW-OFF_GPIO_O (Output), LVCMOS25_4mA_SLEW-ON_GPIO_O (Output), LVCMOS25_4mA_SLEW-OFF_GPIO_O (Output), LVCMOS25_6mA_SLEW-ON_GPIO_O (Output), LVCMOS25_6mA_SLEW-OFF_GPIO_O (Output), LVCMOS25_12mA_SLEW-ON_GPIO_O (Output), LVCMOS25_12mA_SLEW-OFF_GPIO_O (Output), LVCMOS25_16mA_SLEW-ON_GPIO_O (Output), LVCMOS25_16mA_SLEW-OFF_GPIO_O (Output), LVCMOS18_8mA_SLEW-OFF_GPIO_O (Output), LVCMOS18_2mA_SLEW-OFF_GPIO_O (Output), LVCMOS18_4mA_SLEW-OFF_GPIO_O (Output), LVCMOS18_6mA_SLEW-OFF_GPIO_O (Output), LVCMOS18_10mA_SLEW-OFF_GPIO_O (Output), LVCMOS18_12mA_SLEW-OFF_GPIO_O (Output), LVCMOS15_8mA_SLEW-OFF_GPIO_O (Output), LVCMOS15_2mA_SLEW-OFF_GPIO_O (Output), LVCMOS15_4mA_SLEW-OFF_GPIO_O (Output), LVCMOS15_6mA_SLEW-OFF_GPIO_O (Output), LVCMOS15_10mA_SLEW-OFF_GPIO_O (Output), LVCMOS12_8mA_SLEW-OFF_GPIO_O (Output), LVCMOS12_2mA_SLEW-OFF_GPIO_O (Output), LVCMOS12_4mA_SLEW-OFF_GPIO_O (Output), LVCMOS12_6mA_SLEW-OFF_GPIO_O (Output), SSTL25_C1_80ohm_SLEW-OFF_GPIO_O (Output), SSTL25_C1_120ohm_SLEW-OFF_GPIO_O (Output), SSTL25_C1_60ohm_SLEW-OFF_GPIO_O (Output), SSTL25_C1_48ohm_SLEW-OFF_GPIO_O (Output), SSTL25_C2_48ohm_SLEW-OFF_GPIO_O (Output), SSTL25_C2_60ohm_SLEW-OFF_GPIO_O (Output), SSTL25_C2_40ohm_SLEW-OFF_GPIO_O (Output), SSTL25_C2_34ohm_SLEW-OFF_GPIO_O (Output), SSTL18_C1_60ohm_SLEW-OFF_GPIO_O (Output), SSTL18_C1_80ohm_SLEW-OFF_GPIO_O (Output), SSTL18_C1_48ohm_SLEW-OFF_GPIO_O (Output), SSTL18_C1_40ohm_SLEW-OFF_GPIO_O (Output), SSTL18_C2_40ohm_SLEW-OFF_GPIO_O (Output), SSTL18_C2_48ohm_SLEW-OFF_GPIO_O (Output), SSTL18_C2_34ohm_SLEW-OFF_GPIO_O (Output), SSTL18_C2_30ohm_SLEW-OFF_GPIO_O (Output), SSTL15_C1_40ohm_SLEW-OFF_GPIO_O (Output), SSTL15_C1_48ohm_SLEW-OFF_GPIO_O (Output), SSTL15_C2_34ohm_SLEW-OFF_GPIO_O (Output), SSTL15_C2_30ohm_SLEW-OFF_GPIO_O (Output), SSTL15_C2_27ohm_SLEW-OFF_GPIO_O (Output), HSUL18_C1_55ohm_SLEW-OFF_GPIO_O (Output), HSUL18_C1_60ohm_SLEW-OFF_GPIO_O (Output), HSUL18_C1_40ohm_SLEW-OFF_GPIO_O (Output), HSUL18_C1_34ohm_SLEW-OFF_GPIO_O (Output), HSUL18_C2_25ohm_SLEW-OFF_GPIO_O (Output), HSUL18_C2_30ohm_SLEW-OFF_GPIO_O (Output)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
